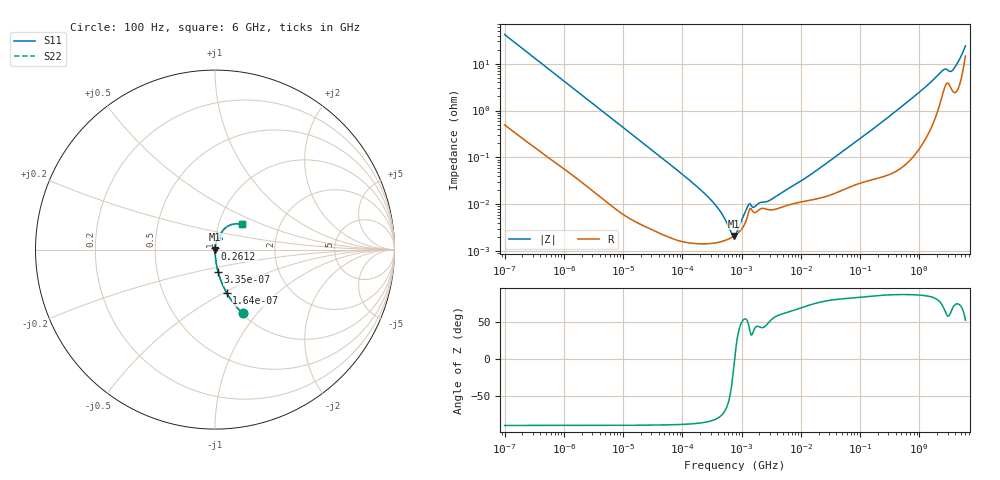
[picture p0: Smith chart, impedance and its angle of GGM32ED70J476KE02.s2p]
!Murata Part Number: GGM32ED70J476KE02
!These Parameters are Measured in Series Mode Connection
!Data Generated on Mar 13, 2026
!  o--ll--o
!Port1  Port2
!  o------o
!Operation Temp=25[degC], DC Bias Voltage=0[V]
!Freq. Start=100[Hz] Stop=6[GHz] 401[Steps]
# Hz S RI R 50
!Freq.(Hz) S11(Real) S11(Imag) S21(Real) S21(Imag) S12(Real) S12(Imag) S22(Real) S22(Imag)
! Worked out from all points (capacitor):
!   401 points, 100 Hz to 6 GHz, reference 50 ohm
!   read as one part in series: C = 37.7 uF near 109 Hz
!   lowest |Z| = 2.12 mohm at 740.7 kHz (marker M1)
!   series resonance near 762.7 kHz, so ESL is about 1.2 nH
!   S11 on the Smith chart (normalised r, x): 100 Hz: 1.01, -0.84; 164 Hz: 1.01, -0.52; 335 Hz: 1.00, -0.25; 261.2 MHz: 1.00, +0.01; 6 GHz: 1.29, +0.38
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100  0.1534 -0.3546  0.8466 0.3546  0.8466 0.3546  0.1534 -0.3546
164  0.065 -0.2407  0.935 0.2407  0.935 0.2407  0.065 -0.2407
335  0.0173 -0.1244  0.9827 0.1244  0.9827 0.1244  0.0173 -0.1244
2008  0.000755 -0.0215  0.9992 0.0215  0.9992 0.0215  0.000755 -0.0215
40335  2.56e-05 -0.00109  1 0.00109  1 0.00109  2.56e-05 -0.00109
161617  1.46e-05 -0.000263  1 0.000263  1 0.000263  1.46e-05 -0.000263
345986  1.49e-05 -0.000103  1 0.000103  1 0.000103  1.49e-05 -0.000103
395726  1.53e-05 -8.27e-05  1 8.27e-05  1 8.27e-05  1.53e-05 -8.27e-05
740679  2.09e-05 -3.5e-06  1 3.5e-06  1 3.5e-06  2.09e-05 -3.5e-06
774597  2.17e-05 1.9e-06  1 -1.9e-06  1 -1.9e-06  2.17e-05 1.9e-06
1734173  6.75e-05 6.38e-05  0.9999 -6.38e-05  0.9999 -6.38e-05  6.75e-05 6.38e-05
2837864  7.68e-05 8.88e-05  0.9999 -8.88e-05  0.9999 -8.88e-05  7.68e-05 8.88e-05
1.555665e7  0.000125 0.000437  0.9999 -0.000437  0.9999 -0.000437  0.000125 0.000437
2.61201e8  0.000437 0.00631  0.9996 -0.00631  0.9996 -0.00631  0.000437 0.00631
3.124326e8  0.000488 0.00754  0.9995 -0.00754  0.9995 -0.00754  0.000488 0.00754
1.094528e9  0.00253 0.027  0.9975 -0.027  0.9975 -0.027  0.00253 0.027
2.450438e9  0.025 0.0645  0.975 -0.0645  0.975 -0.0645  0.025 0.0645
2.802721e9  0.0387 0.0632  0.9613 -0.0632  0.9613 -0.0632  0.0387 0.0632
3.352442e9  0.0342 0.0562  0.9658 -0.0562  0.9658 -0.0562  0.0342 0.0562
3.666503e9  0.0295 0.0645  0.9705 -0.0645  0.9705 -0.0645  0.0295 0.0645
4.796499e9  0.0476 0.1108  0.9524 -0.1108  0.9524 -0.1108  0.0476 0.1108
6e9  0.1508 0.1414  0.8492 -0.1414  0.8492 -0.1414  0.1508 0.1414
